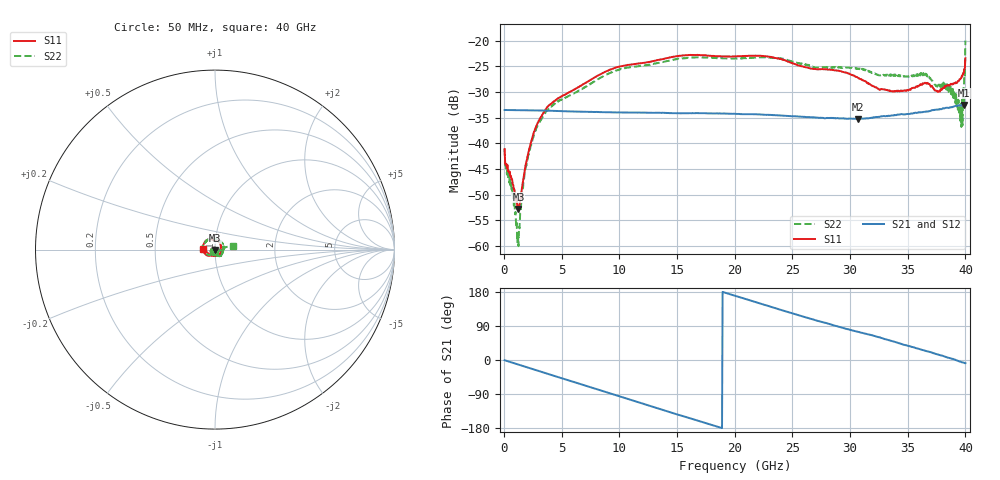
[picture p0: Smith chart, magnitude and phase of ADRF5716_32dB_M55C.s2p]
! Device: ADRF5716
! Description: 30GHz 2-Bit Digital Attenuator
! Frequency: 100 MHz – 30 GHz
! Ports:
! ATTIN  = Port 1
! ATTOUT = Port 2
! State: 32 dB Attenuation selected
! Supply Voltage:
! VDD  =  +3.30 Volts
! VSS  =  -3.30 Volts
! Control Voltages:
! D5 = 0V, D6 = 3.3V
! Temperature = -55 C
! Data: Data was collected using a calibrated network analyzer.
!  The reference plane is the package pins of ADRF5716 switch.
! Note: Analog Devices supplies this data as a sample of measured data for this product.
!  Your particular data for this product may vary.
!  Analog Devices reserves the right to change this data at anytime
# HZ S DB R 50
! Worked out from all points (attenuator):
!   800 points, 50 MHz to 40 GHz, reference 50 ohm
!   highest |S21| = -32.51 dB at 39.9 GHz (marker M1); lowest = -35.2 dB at 30.65 GHz (marker M2)
!   lowest |S11| = -52.8 dB at 1.25 GHz (marker M3), VSWR 1.00, Z = 49.9 - j0.174 ohm
!   |S11| at or under -10 dB: start of sweep to end of sweep
!   |S22| runs from -60.0 to -20.0 dB; largest |S21 - S12| = 0
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5e7  -41.13 -136.3  -33.52 -0.5  -33.52 -0.5  -41.09 -134.7
7e8  -47.02 176.7  -33.53 -6.9  -33.53 -6.9  -48.48 168.4
1.05e9  -51.10 -160.2  -33.54 -10.2  -33.54 -10.2  -56.19 -174.9
1.25e9  -52.78 -130.3  -33.56 -12.1  -33.56 -12.1  -60.02 -110.8
1.9e9  -43.94 -87.4  -33.56 -18.3  -33.56 -18.3  -44.32 -76.5
2.9e9  -36.09 -91.8  -33.59 -27.9  -33.59 -27.9  -36.58 -88.3
4.05e9  -32.34 -107.5  -33.66 -39.1  -33.66 -39.1  -32.87 -107.2
6.75e9  -28.64 -124.3  -33.83 -64.7  -33.83 -64.7  -29.45 -126.8
9.65e9  -25.27 -143.2  -33.98 -92.5  -33.98 -92.5  -25.87 -146.9
1.34e10  -23.74 -166.0  -34.04 -128.3  -34.04 -128.3  -24.32 -172.7
2.005e10  -23.08 151.5  -34.27 169.2  -34.27 169.2  -23.46 140.4
2.305e10  -23.16 127.4  -34.45 141.3  -34.45 141.3  -23.33 116.1
2.67e10  -25.47 98.0  -34.93 107.9  -34.93 107.9  -25.07 79.3
3.065e10  -27.18 46.8  -35.23 74.6  -35.23 74.6  -25.42 34.5
3.335e10  -29.70 8.4  -34.63 52.3  -34.63 52.3  -26.80 0.0
3.665e10  -28.37 -61.2  -33.79 23.2  -33.79 23.2  -26.58 -50.2
3.76e10  -29.97 -84.3  -33.42 14.6  -33.42 14.6  -28.68 -62.8
3.87e10  -28.50 -110.8  -32.98 4.7  -32.98 4.7  -28.88 -73.6
3.955e10  -27.49 -144.6  -32.64 -4.4  -32.64 -4.4  -35.62 -70.8
3.975e10  -26.85 -156.1  -32.60 -6.3  -32.60 -6.3  -36.48 -29.3
3.99e10  -25.61 -169.6  -32.51 -7.4  -32.51 -7.4  -25.60 7.2
4e10  -23.44 176.6  -32.61 -8.3  -32.61 -8.3  -19.97 13.1
